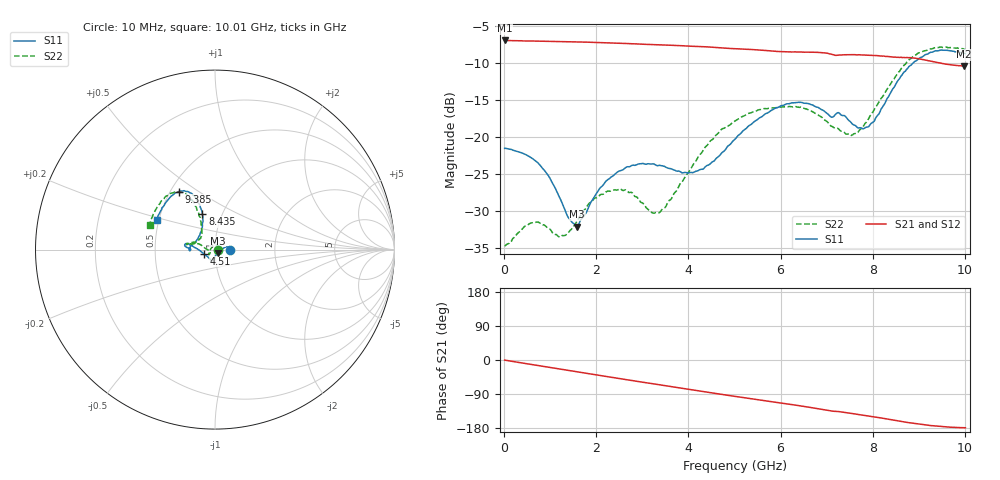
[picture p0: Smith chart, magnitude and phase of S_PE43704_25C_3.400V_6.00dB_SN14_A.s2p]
! Device ID: PE43704
! Dir: z:\PE43704\PE43704_Char_1_20130516\PE43704\AMB\3p400V\6p00dB
! Serial: 14
! Insertion: A
! Impedance: 50 ohm
! Temp: Amb
! VDD: 3.400V
! Attenuation Step: 6.00dB
! IDD: 1.140975e-01mA
#  Hz  S  RI  R  50
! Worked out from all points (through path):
!   401 points, 10 MHz to 10.01 GHz, reference 50 ohm
!   highest |S21| = -6.98 dB at 10 MHz (marker M1); lowest = -10.5 dB at 9.985 GHz (marker M2)
!   group delay of S21, straight-line fit = 51.1 ps
!   lowest |S11| = -32.2 dB at 1.585 GHz (marker M3), VSWR 1.05, Z = 51.6 - j1.96 ohm
!   |S11| at or under -10 dB: start of sweep to 8.881 GHz
!   |S22| runs from -34.8 to -7.9 dB; largest |S21 - S12| = 0.0032
!   S11 on the Smith chart (normalised r, x): 10 MHz: 1.18, +0.00; 4.51 GHz: 0.88, -0.04; 8.435 GHz: 0.81, +0.34; 9.385 GHz: 0.55, +0.42; 10.01 GHz: 0.49, +0.19
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1e7  0.0834 6.61e-05  0.4476 -0.0017  0.4479 -0.0017  0.0182 0.000535
4.85e8  0.074 0.0133  0.4379 -0.075  0.4379 -0.0749  0.0131 0.0214
7.6e8  0.0635 0.0149  0.4276 -0.1156  0.4276 -0.1155  0.00524 0.0257
1.235e9  0.037 -0.00021  0.4008 -0.182  0.401 -0.1819  -0.0144 0.0156
1.585e9  0.0157 -0.019  0.3741 -0.227  0.3742 -0.2268  -0.0267 -0.00161
1.685e9  0.0112 -0.0256  0.3656 -0.2393  0.3656 -0.2391  -0.0299 -0.00668
2.085e9  -0.00385 -0.045  0.327 -0.2835  0.3272 -0.2835  -0.0342 -0.0217
2.51e9  -0.0127 -0.0573  0.2803 -0.3238  0.2805 -0.3238  -0.0348 -0.0277
3.36e9  -0.0212 -0.0603  0.1756 -0.3795  0.1761 -0.3793  -0.0284 -0.0112
4.035e9  -0.0401 -0.0408  0.0857 -0.4005  0.0863 -0.4007  -0.0584 0.0108
4.51e9  -0.0634 -0.0224  0.0217 -0.4026  0.0219 -0.4027  -0.0901 0.0306
5.01e9  -0.0961 0.00203  -0.0411 -0.3915  -0.041 -0.3919  -0.1236 0.0319
5.935e9  -0.1539 0.0332  -0.1434 -0.3487  -0.1425 -0.3499  -0.1543 0.0332
6.685e9  -0.1635 0.016  -0.2191 -0.3013  -0.2194 -0.3011  -0.1438 0.0348
7.585e9  -0.1134 0.0399  -0.2824 -0.2215  -0.2819 -0.221  -0.079 0.0681
7.935e9  -0.083 0.0862  -0.3029 -0.1865  -0.3028 -0.1872  -0.0741 0.1154
8.36e9  -0.068 0.1786  -0.3192 -0.1375  -0.3189 -0.1385  -0.0907 0.2007
8.435e9  -0.0702 0.199  -0.3219 -0.1279  -0.321 -0.1285  -0.0995 0.2185
8.86e9  -0.1103 0.292  -0.3319 -0.0784  -0.3298 -0.0795  -0.1593 0.307
9.385e9  -0.2033 0.3224  -0.3168 -0.0309  -0.3179 -0.0294  -0.2569 0.3059
9.985e9  -0.3197 0.1773  -0.3 -0.00675  -0.3015 -0.00563  -0.3607 0.1471
1.001e10  -0.3249 0.1667  -0.3011 -0.00639  -0.303 -0.00606  -0.3647 0.1381
